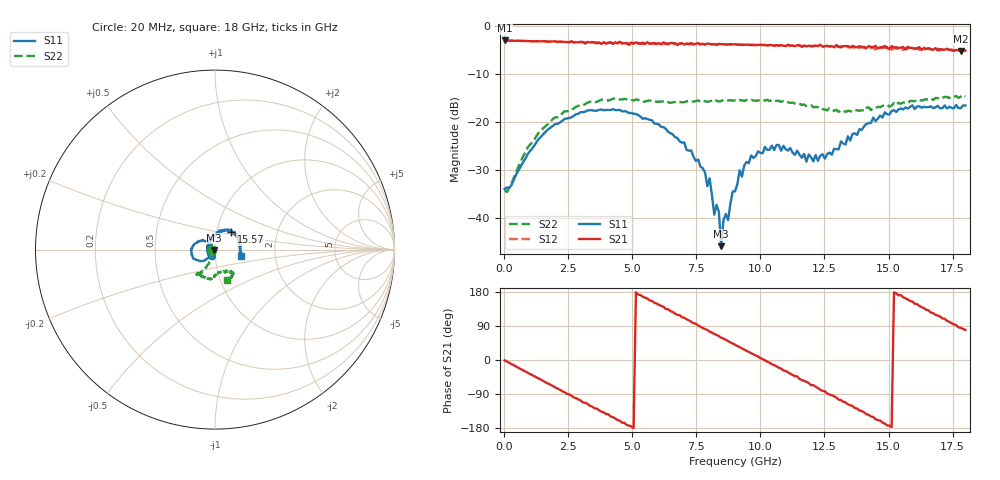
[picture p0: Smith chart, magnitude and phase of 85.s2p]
!Agilent Technologies,N5230A,US43500223,A.07.50.48
!Agilent N5230A: A.07.50.48
!Date: Sunday, January 31, 2016 15:12:58
!Correction: S11(Full 2 Port(1,2))
!S21(Full 2 Port(1,2))
!S12(Full 2 Port(1,2))
!S22(Full 2 Port(1,2))
!S2P File: Measurements: S11, S21, S12, S22:
# Hz S  dB  R 50
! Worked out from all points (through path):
!   201 points, 20 MHz to 18 GHz, reference 50 ohm
!   highest |S21| = -3.11 dB at 20 MHz (marker M1); lowest = -5.3 dB at 17.82 GHz (marker M2)
!   group delay of S21, straight-line fit = 98.7 ps
!   lowest |S11| = -45.9 dB at 8.471 GHz (marker M3), VSWR 1.01, Z = 49.5 - j0.136 ohm
!   |S11| at or under -10 dB: start of sweep to end of sweep
!   |S22| runs from -34.7 to -14.5 dB; largest |S21 - S12| = 0.063
!   S11 on the Smith chart (normalised r, x): 20 MHz: 0.96, -0.00; 15.57 GHz: 1.17, +0.24; 18 GHz: 1.33, -0.10
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2e7  -34.05 -178.7  -3.11 -0.8  -3.11 -0.9  -34.28 180.0
1.5483e9  -22.50 -132.5  -3.22 -56.1  -3.25 -56.4  -21.26 -113.2
3.0766e9  -18.04 -155.4  -3.42 -112.2  -3.49 -111.7  -16.61 -121.8
4.515e9  -17.54 177.9  -3.45 -160.1  -3.36 -162.3  -15.39 -125.6
6.0433e9  -20.61 148.5  -3.65 145.2  -3.85 143.5  -15.88 -124.6
6.9423e9  -24.40 134.4  -3.67 112.8  -3.86 112.5  -15.98 -120.8
8.0211e9  -31.83 136.5  -3.82 74.7  -3.91 74.2  -15.79 -119.1
8.2009e9  -39.37 140.0  -3.87 68.5  -3.93 67.7  -15.36 -115.8
8.3807e9  -38.81 -178.3  -3.79 63.0  -3.94 61.3  -15.85 -115.5
8.4706e9  -45.94 -164.2  -3.89 58.9  -3.95 58.0  -15.72 -115.8
8.5605e9  -40.56 -154.7  -3.88 56.8  -3.94 54.9  -15.52 -115.3
8.7403e9  -40.52 -105.8  -3.95 50.2  -3.95 48.4  -15.60 -112.8
9.01e9  -34.55 -103.4  -3.88 40.5  -3.99 38.9  -15.58 -110.5
9.1898e9  -30.13 -95.8  -4.02 34.1  -4.05 32.4  -15.58 -108.3
1.01787e10  -25.27 -99.8  -4.02 -0.9  -4.11 -3.1  -15.60 -99.0
1.20666e10  -28.28 -177.6  -4.33 -66.1  -4.21 -70.2  -17.03 -89.9
1.35949e10  -22.57 97.6  -4.25 -121.3  -4.54 -126.7  -17.95 -73.5
1.50333e10  -18.55 62.9  -4.96 -173.2  -4.74 -178.3  -16.91 -56.5
1.55727e10  -17.49 47.9  -4.49 165.5  -5.09 164.4  -16.02 -52.7
1.67414e10  -17.18 21.7  -5.06 123.6  -4.84 120.3  -15.51 -55.1
1.78202e10  -17.20 -11.2  -5.30 85.0  -5.33 80.5  -14.79 -63.0
1.8e10  -16.66 -14.3  -5.21 79.2  -5.28 74.2  -14.77 -69.1
